FUNCTION_BLOCK FB_LN_IED_LD1_LEDGGIO2 EXTENDS FB_AcsiCommonLogicalNodeClass
VAR_INPUT
	NamPlt: FB_DO_IED_LD1_LEDGGIO2_NamPlt := (sClass:='LPL', bLinkResult:=THIS^.AddDataToContainer(ipData:=NamPlt));
	Beh: FB_DO_IED_LD1_LEDGGIO2_Beh := (sClass:='ENS', bLinkResult:=THIS^.AddDataToContainer(ipData:=Beh));
	Health: FB_DO_IED_LD1_LEDGGIO2_Health := (sClass:='ENS', bLinkResult:=THIS^.AddDataToContainer(ipData:=Health));
	Mod_: FB_DO_IED_LD1_LEDGGIO2_Mod := (sObjectName:='Mod', sClass:='ENC', bLinkResult:=THIS^.AddDataToContainer(ipData:=Mod_));
	AnOut1: FB_DO_IED_LD1_LEDGGIO2_AnOut1 := (sClass:='APC', bLinkResult:=THIS^.AddDataToContainer(ipData:=AnOut1));
	SPCSO1: FB_DO_IED_LD1_LEDGGIO2_SPCSO1 := (sClass:='SPC', bLinkResult:=THIS^.AddDataToContainer(ipData:=SPCSO1));
	DPCSO1: FB_DO_IED_LD1_LEDGGIO2_DPCSO1 := (sClass:='DPC', bLinkResult:=THIS^.AddDataToContainer(ipData:=DPCSO1));
	ISCSO1: FB_DO_IED_LD1_LEDGGIO2_ISCSO1 := (sClass:='INC', bLinkResult:=THIS^.AddDataToContainer(ipData:=ISCSO1));
END_VAR
VAR
END_VAR

END_FUNCTION_BLOCK
